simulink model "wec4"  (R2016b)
settings: Solver=ode4  StartTime=0  StopTime=1000  FixedStep=0.005  MaxStep=0.005  RelTol=1e-3  EnableMultiTasking=on
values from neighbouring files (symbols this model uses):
  arAdaptiveLawData = 1/2*zModelSimple.zModelPto.arFreq.*     zModelSimple.zModelPto.arMagnitude./     cos(zModelSimple.zModelPto.arPhase*pi/180+pi/2)    [IMPACT_Control.m]
  arAdaptiveLawDataX = 1/2*zModelSimpleX.zModelPto.arFreq.*         zModelSimpleX.zModelPto.arMagnitude./         cos(zModelSimpleX.zModelPto.arPhase*pi/180+pi/2)    [IMPACT_Control.m]
  arControllerRampGain = [0,0,1,1]    [IMPACT_Control.m]
  arControllerRampTime = [0 rStartRampTime rStartRampTime+rRampTimeLength 8000]    [IMPACT_Control.m]
  arEkfInitialisation = zeros(1,11)    [IMPACT_Control.m]
  arEkfInitialisationX = zeros(1,11)    [IMPACT_Control.m]
  arFrequency = zModelSimple.zModelPto.arFreq    [IMPACT_Control.m]
  arFrequencyRange = zModelSimple.zModelPto.arFreq    [IMPACT_Control.m]
  arFrequencyX = zModelSimpleX.zModelPto.arFreq    [IMPACT_Control.m]
  arImpedance = 1./zModelSimple.zModelPto.arMagnitude./zModelSimple.zModelPto.arFreq    [IMPACT_Control.m]
  arImpedanceX = 1./zModelSimpleX.zModelPto.arMagnitude./zModelSimpleX.zModelPto.arFreq    [IMPACT_Control.m]
  CentralPTOPreload = -1.6113e+07    (= -16113000)    [wecSimInputFile.m]
  F1 = [4.243 2.375 -12.243]    [wecSimInputFile.m]
  F2 = [4.243 -2.375 -12.243]    [wecSimInputFile.m]
  F3 = [-4.243 -2.375 -12.243]    [wecSimInputFile.m]
  F4 = [-4.243 2.375 -12.243]    [wecSimInputFile.m]
  FC = [0 0 -14]    [wecSimInputFile.m]
  iAdaptiveDamping = 0    [wec4IMPACT_Project.m]    (also in IMPACT_Control.m = handles.iAdaptiveDamping; wec1_IMPACT_Project.m; wec2_IMPACT_Project.m; wec3_IMPACT_Project.m)
  iControlType = 2    [wec4IMPACT_Project.m]    (also in IMPACT_Control.m = handles.iControlType; wec1_IMPACT_Project.m = 1; wec2_IMPACT_Project.m = 1; wec3_IMPACT_Project.m = 1)
  iPtoPositionConstraint = 1    [wec4IMPACT_Project.m]    (also in IMPACT_Control.m = handles.iPtoPositionConstraint; wec1_IMPACT_Project.m = 0; wec2_IMPACT_Project.m; wec3_IMPACT_Project.m)
  iSensorNoise = 0    [IMPACT_Control.m]
  m = m+1    (= 2)    [checkParamFile.m]
  PTOrotation = atan((T1(2)-F1(2))/(T1(1)-F1(1)))    [wecSimInputFile.m]
  rCogFloater = -8    [wec4_IMPACT_Model.m]    (also in paramInitial.m = get( handles.edit_rCogFloater, 'String' ); wec1_IMPACT_Model.m = -18; wec2_IMPACT_Model.m = -8.5; wec3_IMPACT_Model.m = -0.7)
  rCogSpar = -36.6    [wec4_IMPACT_Model.m]    (also in paramInitial.m = get( handles.edit_rCogSpar, 'String' ); wec3_IMPACT_Model.m = -21.3; wec3_IMPACT_Model2.m = -21.3)
  rDisplacementLimit = 10.000000    (= 10)    [wec4IMPACT_Project.m]    (also in IMPACT_Control.m = getValue(handles.edit_displacementLimit); wec1_IMPACT_Project.m; wec2_IMPACT_Project.m; wec3_IMPACT_Project.m = 3)
  rDisplacementLimitX = 10.000000    (= 10)    [wec4IMPACT_Project.m]    (also in IMPACT_Control.m = getValue(handles.edit_displacementLimitX); wec1_IMPACT_Project.m = 0; wec2_IMPACT_Project.m; wec3_IMPACT_Project.m = 0)
  rGainForAntiWIndUp = tfControllerDiscrete.rGain    [IMPACT_Control.m]
  rGainForAntiWIndUpX = tfControllerXDiscrete.rGain    [IMPACT_Control.m]
  rMaxForcePto = 300000000.000000    (= 300000000)    [wec4IMPACT_Project.m]    (also in IMPACT_Control.m = getValue(handles.edit_maxForcePto); wec1_IMPACT_Project.m = 1e+15; wec2_IMPACT_Project.m = 1e+15; wec3_IMPACT_Project.m = 1000000000)
  rMinForcePto = -300000000.000000    (= -300000000)    [wec4IMPACT_Project.m]    (also in IMPACT_Control.m = getValue(handles.edit_minForcePto); wec1_IMPACT_Project.m = -1e+15; wec2_IMPACT_Project.m = -1e+15; wec3_IMPACT_Project.m = -1000000000)
  rMooringX = 20000    [wec4_IMPACT_Model.m]    (also in paramInitial.m = get( handles.edit_rMooringX, 'String' ); wec3_IMPACT_Model.m = 10000; wec3_IMPACT_Model2.m = 10000)
  rMooringZ = 10000    [wec4_IMPACT_Model.m]    (also in paramInitial.m = get( handles.edit_rMooringZ, 'String' ); wec3_IMPACT_Model.m = 0; wec3_IMPACT_Model2.m = 0)
  rOutputSampleTime = 0.010000    (= 0.01)    [wec4IMPACT_Project.m]    (also in IMPACT_Control.m = getValue(handles.edit_outputSampleTime); wec1_IMPACT_Project.m; wec2_IMPACT_Project.m; wec3_IMPACT_Project.m)
  rPassiveDampingGain = -604830.000000    (= -604830)    [wec4IMPACT_Project.m]    (also in IMPACT_Control.m = getValue(handles.edit_gainPLD); wec1_IMPACT_Project.m = -214018.1537; wec2_IMPACT_Project.m = -1948070; wec3_IMPACT_Project.m = -519390)
  rPassiveDampingGainX = -278660.000000    (= -278660)    [wec4IMPACT_Project.m]    (also in IMPACT_Control.m = getValue(handles.edit_gainPLDX); wec1_IMPACT_Project.m = 0; wec2_IMPACT_Project.m = 0; wec3_IMPACT_Project.m = 0)
  rTetherPretension = 1.6113e+07    (= 16113000)    [wec4_IMPACT_Model.m]    (also in paramInitial.m = get( handles.edit_rTetherPretension, 'String' ); wec3_IMPACT_Model.m = 0; wec3_IMPACT_Model2.m = 0)
  rTetherSpring = 500000    [wec4_IMPACT_Model.m]    (also in paramInitial.m = get( handles.edit_rTetherSpring, 'String' ); wec3_IMPACT_Model.m = 0; wec3_IMPACT_Model2.m = 0)
  rUpperFrequencyLimit = EKFFloater.upperFreq    [IMPACT_Control.m]
  rXf = 4.243    [wec4AdditionalParams.m]
  rXs = 16.075    [wec4AdditionalParams.m]
  rYf = 2.375    [wec4AdditionalParams.m]
  rYs = 16.075    [wec4AdditionalParams.m]
  rZf = 4.243    [wec4AdditionalParams.m]
  rZs = 2.4350    (= 2.435)    [wec4AdditionalParams.m]
  rZTetherF = 6    [wec4AdditionalParams.m]
  rZTetherS = 2.4350    (= 2.435)    [wec4AdditionalParams.m]
  s = tf('s')    [wec4_IMPACT_Model.m]    (also in IMPACT_Control.m; wec1_IMPACT_Model.m; wec2_IMPACT_Model.m; wec3_IMPACT_Model.m)
  SidePTO1Preload = PreloadPTOCorner    (= 0)    [wecSimInputFile.m]
  SidePTO2Preload = PreloadPTOCorner    (= 0)    [wecSimInputFile.m]
  SidePTO3Preload = PreloadPTOCorner    (= 0)    [wecSimInputFile.m]
  SidePTO4Preload = PreloadPTOCorner    (= 0)    [wecSimInputFile.m]
  simu = simulationClass()    [wecSimInputFile.m]
  T1 = [16.075 16.075 -34.165]    [wecSimInputFile.m]
  T2 = [16.075 -16.075 -34.165]    [wecSimInputFile.m]
  T3 = [-16.075 -16.075 -34.165]    [wecSimInputFile.m]
  T4 = [-16.075 16.075 -34.165]    [wecSimInputFile.m]
  TC = [0 0 -34.165]    [wecSimInputFile.m]
  waves = waveClass('irregular')    [wecSimInputFile.m]
  Z = magPhaseToComplex(zModelTf)    [IMPACT_Control.m]
undefined symbols (not defined in the file or in its folder): arControllerDiscreteDen, arControllerDiscreteNum, arControllerDiscreteXDen, arControllerDiscreteXNum, arExcForceFloaterDen, arExcForceFloaterNum, arExcForceFloaterXDen, arExcForceFloaterXNum, arExcForceSparDen, arExcForceSparNum, arExcForceSparXDen, arExcForceSparXNum, arFexcFloaterDen, arFexcFloaterNum, arFexcFloaterXDen, arFexcFloaterXNum, arFexcSparDen, arFexcSparNum, arFexcSparXDen, arFexcSparXNum, Body, body, constraint, CTTime, deg, Elements, geometry, IRKB, kg, lenJ, mooring, N, pto, rAccelerationGainFloater, rAccelerationGainFloaterX, rAccelerationGainSpar, rAccelerationGainSparX, rad, rBuoyancyGainFloater, rBuoyancyGainFloaterX, rBuoyancyGainSpar, rBuoyancyGainSparX, rDampingGainFloater, rDampingGainFloaterX, rDampingGainSpar, rDampingGainSparX, Rigid, rMaxFocePto, wec4_float, wec4_reactor, WECSim_Lib, X, Y
libraries: nesl_utility x380, sm_lib x170, vrlib x91, simulink x12, WECSim_Lib x4
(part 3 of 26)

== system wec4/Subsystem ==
  Vel floater 6x1 : Inport
  Vel Spar 6x1 : Inport  Port=2
  Selector1 : Selector  InputPortWidth=6  IndexOptions=Index vector (dialog)  Indices=3  OutputSizes=1
  Selector18 : Selector  InputPortWidth=6  IndexOptions=Index vector (dialog)  Indices=1  OutputSizes=1
  Selector2 : Selector  InputPortWidth=6  IndexOptions=Index vector (dialog)  Indices=3  OutputSizes=1
  Selector3 : Selector  InputPortWidth=6  IndexOptions=Index vector (dialog)  Indices=1  OutputSizes=1
  Sum5 : Sum  Inputs=|+-
  Sum6 : Sum  Inputs=|+-
  "Rel. vel. X " : Outport
  Rel. vel. Z : Outport  Port=2
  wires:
  Selector1/1 -> Sum6/1
  Selector2/1 -> Sum6/2
  Vel floater 6x1/1 -> Selector1/1, Selector18/1
  Selector3/1 -> Sum5/2
  Vel Spar 6x1/1 -> Selector2/1, Selector3/1
  Selector18/1 -> Sum5/1
  Sum5/1 -> "Rel. vel. X "/1
  Sum6/1 -> Rel. vel. Z/1

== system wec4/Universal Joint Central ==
  Assignment : Assignment  DiagnosticForDimensions=Warning  IndexOptions=Index vector (dialog)  Indices=[4 5]  OutputSizes=1
  Assignment1 : Assignment  DiagnosticForDimensions=Warning  IndexOptions=Index vector (dialog)  Indices=[4 5]  OutputSizes=1
  Assignment2 : Assignment  DiagnosticForDimensions=Warning  IndexOptions=Index vector (dialog)  Indices=[4 5]  OutputSizes=1
  CONSTRAINT Universal Joint : sm_lib/Joints/Universal Joint  SenseConstraintForce=on  SenseConstraintForceX=off  SenseConstraintForceY=off  SenseConstraintForceZ=off  SenseConstraintTorque=on  SenseConstraintTorqueX=off  SenseConstraintTorqueY=off  SenseConstraintTorqueZ=off  SenseTotalForce=off  SenseTotalForceX=off  SenseTotalForceY=off  SenseTotalForceZ=off  SenseTotalTorque=off  SenseTotalTorqueX=off  SenseTotalTorqueY=off  SenseTotalTorqueZ=off  CompositeWrenchDir=BaseOnFollower  CompositeWrenchFrame=BaseFrame  RxEquilibriumPosition=0  RxEquilibriumPositionUnits=deg  RxSpringStiffness=0  RxSpringStiffnessUnits=N*m/deg  RxDampingCoefficient=0  RxDampingCoefficientUnits=N*m/(deg/s)  RxTorqueActuationMode=NoTorque  RxMotionActuationMode=ComputedMotion  RxSensePosition=on  RxSenseVelocity=on  RxSenseAcceleration=on  RxSenseTorqueForce=off  RxPositionTargetSpecify=off  RxPositionTargetPriority=High  RxPositionTargetValue=0  RxPositionTargetValueUnits=deg  RxVelocityTargetSpecify=off  RxVelocityTargetPriority=High  RxVelocityTargetValue=0  RxVelocityTargetValueUnits=deg/s  RyEquilibriumPosition=0  RyEquilibriumPositionUnits=deg  RySpringStiffness=0  RySpringStiffnessUnits=N*m/deg  RyDampingCoefficient=0  RyDampingCoefficientUnits=N*m/(deg/s)  RyTorqueActuationMode=NoTorque  RyMotionActuationMode=ComputedMotion  RySensePosition=on  RySenseVelocity=on  RySenseAcceleration=on  RySenseTorqueForce=off  RyPositionTargetSpecify=off  RyPositionTargetPriority=High  RyPositionTargetValue=0  RyPositionTargetValueUnits=deg  RyVelocityTargetSpecify=off  RyVelocityTargetPriority=High  RyVelocityTargetValue=0  RyVelocityTargetValueUnits=deg/s
  Constant : Constant  Value=[0 0 0 0 0 0]
  Constant1 : Constant  Value=[0 0 0 0 0 0]
  Constant2 : Constant  Value=[0 0 0 0 0 0]
  Mux{,2..4} (4 alike) : Mux  Inputs=2
  Mux1 : Mux
  PS-Simulink Converter{1..5,7,9,11} (8 alike) : nesl_utility/PS-Simulink Converter  PhysicalDomain=network_engine_domain  SubClassName=ps_output  LeftPortType=input  RightPortType=output  PseudoPeriodic=off  Frequencies=[]  Unit=1  AffineConversion=off
  Rigid Transform (Position) : sm_lib/Frames and Transforms/Rigid Transform  TranslationMethod=Cartesian  TranslationStandardOffset=0  TranslationLengthUnit=m  TranslationStandardAxis=+Z  TranslationCartesianOffset=constraint.initDisp.initLinDisp+constraint.loc  TranslationROffset=0  TranslationROffsetUnits=m  TranslationZOffset=0  TranslationZOffsetUnits=m  TranslationThetaOffset=0  TranslationThetaOffsetUnits=deg  RotationMethod=None  RotationAngleUnits=rad  RotationStandardAxis=+Y  RotationAngle=0  RotationArbitraryAxis=[0 1 0]  FollAlignAxisA=+X  BaseAlignAxisA=+Y  FollAlignAxisB=+Y  BaseAlignAxisB=+Z  RotationSequenceAxes=FollowerAxes  RotationSequence=XYX  RotationSequenceAngles=[0 0 0]  RotationSequenceAnglesUnits=deg  RotationMatrix=[1 0 0; 0 1 0; 0 0 1]
  Rigid Transform (Position)1 : sm_lib/Frames and Transforms/Rigid Transform  TranslationMethod=Cartesian  TranslationStandardOffset=0  TranslationLengthUnit=m  TranslationStandardAxis=+Z  TranslationCartesianOffset=constraint.initDisp.initLinDisp+constraint.loc  TranslationROffset=0  TranslationROffsetUnits=m  TranslationZOffset=0  TranslationZOffsetUnits=m  TranslationThetaOffset=0  TranslationThetaOffsetUnits=deg  RotationMethod=None  RotationAngleUnits=rad  RotationStandardAxis=+Y  RotationAngle=0  RotationArbitraryAxis=[0 1 0]  FollAlignAxisA=+X  BaseAlignAxisA=+Y  FollAlignAxisB=+Y  BaseAlignAxisB=+Z  RotationSequenceAxes=FollowerAxes  RotationSequence=XYX  RotationSequenceAngles=[0 0 0]  RotationSequenceAnglesUnits=deg  RotationMatrix=[1 0 0; 0 1 0; 0 0 1]
  Rigid Transform (Orientation) : sm_lib/Frames and Transforms/Rigid Transform  TranslationMethod=None  TranslationStandardOffset=0  TranslationLengthUnit=m  TranslationStandardAxis=+Z  TranslationCartesianOffset=constraint.loc  TranslationROffset=0  TranslationROffsetUnits=m  TranslationZOffset=0  TranslationZOffsetUnits=m  TranslationThetaOffset=0  TranslationThetaOffsetUnits=deg  RotationMethod=RotationMatrix  RotationAngleUnits=rad  RotationStandardAxis=+Y  RotationAngle=0  RotationArbitraryAxis=[0 1 0]  FollAlignAxisA=+X  BaseAlignAxisA=+Y  FollAlignAxisB=+Y  BaseAlignAxisB=+Z  RotationSequenceAxes=FollowerAxes  RotationSequence=XYX  RotationSequenceAngles=[0 0 0]  RotationSequenceAnglesUnits=deg  RotationMatrix=constraint.orientation.rotationMatrix
  Rigid Transform (Orientation)1 : sm_lib/Frames and Transforms/Rigid Transform  TranslationMethod=None  TranslationStandardOffset=0  TranslationLengthUnit=m  TranslationStandardAxis=+Z  TranslationCartesianOffset=constraint.loc  TranslationROffset=0  TranslationROffsetUnits=m  TranslationZOffset=0  TranslationZOffsetUnits=m  TranslationThetaOffset=0  TranslationThetaOffsetUnits=deg  RotationMethod=RotationMatrix  RotationAngleUnits=rad  RotationStandardAxis=+Y  RotationAngle=0  RotationArbitraryAxis=[0 1 0]  FollAlignAxisA=+X  BaseAlignAxisA=+Y  FollAlignAxisB=+Y  BaseAlignAxisB=+Z  RotationSequenceAxes=FollowerAxes  RotationSequence=XYX  RotationSequenceAngles=[0 0 0]  RotationSequenceAnglesUnits=deg  RotationMatrix=constraint.orientation.rotationMatrix
  output : ToWorkspace  VariableName=constraint2_out  SaveFormat=Structure With Time  SampleTime=-1
  F : PMIOPort  Port=1  Side=Right
  B : PMIOPort  Port=2  Side=Left
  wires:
  PS-Simulink Converter4/1 -> Mux/2
  PS-Simulink Converter3/1 -> Mux/1
  Mux3/1 -> Assignment1/2
  Mux4/1 -> Assignment/2
  Constant/1 -> Assignment/1
  Constant1/1 -> Assignment1/1
  Constant2/1 -> Assignment2/1
  Assignment2/1 -> Mux1/3  "acceleration"
  Assignment1/1 -> Mux1/2  "velocity"
  Assignment/1 -> Mux1/1  "position"
  Mux/1 -> Mux1/4  "Constraint Forces"
  Mux1/1 -> output/1
  PS-Simulink Converter5/1 -> Mux2/2
  Mux2/1 -> Assignment2/2
  PS-Simulink Converter2/1 -> Mux3/2
  PS-Simulink Converter9/1 -> Mux3/1
  PS-Simulink Converter11/1 -> Mux4/2
  PS-Simulink Converter1/1 -> Mux4/1
  PS-Simulink Converter7/1 -> Mux2/1
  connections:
  Rigid Transform (Position)1/LConn1 -- F/RConn1
  Rigid Transform (Position)1/RConn1 -- Rigid Transform (Orientation)1/LConn1
  Rigid Transform (Orientation)/RConn1 -- CONSTRAINT Universal Joint/LConn1
  Rigid Transform (Position)/RConn1 -- Rigid Transform (Orientation)/LConn1
  Rigid Transform (Position)/LConn1 -- B/RConn1
  CONSTRAINT Universal Joint/RConn8 -- PS-Simulink Converter3/LConn1
  PS-Simulink Converter4/LConn1 -- CONSTRAINT Universal Joint/RConn9
  PS-Simulink Converter1/LConn1 -- CONSTRAINT Universal Joint/RConn2
  PS-Simulink Converter11/LConn1 -- CONSTRAINT Universal Joint/RConn5
  PS-Simulink Converter9/LConn1 -- CONSTRAINT Universal Joint/RConn3
  PS-Simulink Converter7/LConn1 -- CONSTRAINT Universal Joint/RConn4
  PS-Simulink Converter2/LConn1 -- CONSTRAINT Universal Joint/RConn6
  PS-Simulink Converter5/LConn1 -- CONSTRAINT Universal Joint/RConn7
  CONSTRAINT Universal Joint/RConn1 -- Rigid Transform (Orientation)1/RConn1

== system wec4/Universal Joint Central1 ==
  Assignment : Assignment  DiagnosticForDimensions=Warning  IndexOptions=Index vector (dialog)  Indices=[4 5]  OutputSizes=1
  Assignment1 : Assignment  DiagnosticForDimensions=Warning  IndexOptions=Index vector (dialog)  Indices=[4 5]  OutputSizes=1
  Assignment2 : Assignment  DiagnosticForDimensions=Warning  IndexOptions=Index vector (dialog)  Indices=[4 5]  OutputSizes=1
  CONSTRAINT Universal Joint : sm_lib/Joints/Universal Joint  SenseConstraintForce=on  SenseConstraintForceX=off  SenseConstraintForceY=off  SenseConstraintForceZ=off  SenseConstraintTorque=on  SenseConstraintTorqueX=off  SenseConstraintTorqueY=off  SenseConstraintTorqueZ=off  SenseTotalForce=off  SenseTotalForceX=off  SenseTotalForceY=off  SenseTotalForceZ=off  SenseTotalTorque=off  SenseTotalTorqueX=off  SenseTotalTorqueY=off  SenseTotalTorqueZ=off  CompositeWrenchDir=BaseOnFollower  CompositeWrenchFrame=BaseFrame  RxEquilibriumPosition=0  RxEquilibriumPositionUnits=deg  RxSpringStiffness=0  RxSpringStiffnessUnits=N*m/deg  RxDampingCoefficient=0  RxDampingCoefficientUnits=N*m/(deg/s)  RxTorqueActuationMode=NoTorque  RxMotionActuationMode=ComputedMotion  RxSensePosition=on  RxSenseVelocity=on  RxSenseAcceleration=on  RxSenseTorqueForce=off  RxPositionTargetSpecify=off  RxPositionTargetPriority=High  RxPositionTargetValue=0  RxPositionTargetValueUnits=deg  RxVelocityTargetSpecify=off  RxVelocityTargetPriority=High  RxVelocityTargetValue=0  RxVelocityTargetValueUnits=deg/s  RyEquilibriumPosition=0  RyEquilibriumPositionUnits=deg  RySpringStiffness=0  RySpringStiffnessUnits=N*m/deg  RyDampingCoefficient=0  RyDampingCoefficientUnits=N*m/(deg/s)  RyTorqueActuationMode=NoTorque  RyMotionActuationMode=ComputedMotion  RySensePosition=on  RySenseVelocity=on  RySenseAcceleration=on  RySenseTorqueForce=off  RyPositionTargetSpecify=off  RyPositionTargetPriority=High  RyPositionTargetValue=0  RyPositionTargetValueUnits=deg  RyVelocityTargetSpecify=off  RyVelocityTargetPriority=High  RyVelocityTargetValue=0  RyVelocityTargetValueUnits=deg/s
  Constant : Constant  Value=[0 0 0 0 0 0]
  Constant1 : Constant  Value=[0 0 0 0 0 0]
  Constant2 : Constant  Value=[0 0 0 0 0 0]
  Mux{,2..4} (4 alike) : Mux  Inputs=2
  Mux1 : Mux
  PS-Simulink Converter{1..5,7,9,11} (8 alike) : nesl_utility/PS-Simulink Converter  PhysicalDomain=network_engine_domain  SubClassName=ps_output  LeftPortType=input  RightPortType=output  PseudoPeriodic=off  Frequencies=[]  Unit=1  AffineConversion=off
  Rigid Transform (Position) : sm_lib/Frames and Transforms/Rigid Transform  TranslationMethod=Cartesian  TranslationStandardOffset=0  TranslationLengthUnit=m  TranslationStandardAxis=+Z  TranslationCartesianOffset=constraint.initDisp.initLinDisp+constraint.loc  TranslationROffset=0  TranslationROffsetUnits=m  TranslationZOffset=0  TranslationZOffsetUnits=m  TranslationThetaOffset=0  TranslationThetaOffsetUnits=deg  RotationMethod=None  RotationAngleUnits=rad  RotationStandardAxis=+Y  RotationAngle=0  RotationArbitraryAxis=[0 1 0]  FollAlignAxisA=+X  BaseAlignAxisA=+Y  FollAlignAxisB=+Y  BaseAlignAxisB=+Z  RotationSequenceAxes=FollowerAxes  RotationSequence=XYX  RotationSequenceAngles=[0 0 0]  RotationSequenceAnglesUnits=deg  RotationMatrix=[1 0 0; 0 1 0; 0 0 1]
  Rigid Transform (Position)1 : sm_lib/Frames and Transforms/Rigid Transform  TranslationMethod=Cartesian  TranslationStandardOffset=0  TranslationLengthUnit=m  TranslationStandardAxis=+Z  TranslationCartesianOffset=constraint.initDisp.initLinDisp+constraint.loc  TranslationROffset=0  TranslationROffsetUnits=m  TranslationZOffset=0  TranslationZOffsetUnits=m  TranslationThetaOffset=0  TranslationThetaOffsetUnits=deg  RotationMethod=None  RotationAngleUnits=rad  RotationStandardAxis=+Y  RotationAngle=0  RotationArbitraryAxis=[0 1 0]  FollAlignAxisA=+X  BaseAlignAxisA=+Y  FollAlignAxisB=+Y  BaseAlignAxisB=+Z  RotationSequenceAxes=FollowerAxes  RotationSequence=XYX  RotationSequenceAngles=[0 0 0]  RotationSequenceAnglesUnits=deg  RotationMatrix=[1 0 0; 0 1 0; 0 0 1]
  Rigid Transform (Orientation) : sm_lib/Frames and Transforms/Rigid Transform  TranslationMethod=None  TranslationStandardOffset=0  TranslationLengthUnit=m  TranslationStandardAxis=+Z  TranslationCartesianOffset=constraint.loc  TranslationROffset=0  TranslationROffsetUnits=m  TranslationZOffset=0  TranslationZOffsetUnits=m  TranslationThetaOffset=0  TranslationThetaOffsetUnits=deg  RotationMethod=RotationMatrix  RotationAngleUnits=rad  RotationStandardAxis=+Y  RotationAngle=0  RotationArbitraryAxis=[0 1 0]  FollAlignAxisA=+X  BaseAlignAxisA=+Y  FollAlignAxisB=+Y  BaseAlignAxisB=+Z  RotationSequenceAxes=FollowerAxes  RotationSequence=XYX  RotationSequenceAngles=[0 0 0]  RotationSequenceAnglesUnits=deg  RotationMatrix=constraint.orientation.rotationMatrix
  Rigid Transform (Orientation)1 : sm_lib/Frames and Transforms/Rigid Transform  TranslationMethod=None  TranslationStandardOffset=0  TranslationLengthUnit=m  TranslationStandardAxis=+Z  TranslationCartesianOffset=constraint.loc  TranslationROffset=0  TranslationROffsetUnits=m  TranslationZOffset=0  TranslationZOffsetUnits=m  TranslationThetaOffset=0  TranslationThetaOffsetUnits=deg  RotationMethod=RotationMatrix  RotationAngleUnits=rad  RotationStandardAxis=+Y  RotationAngle=0  RotationArbitraryAxis=[0 1 0]  FollAlignAxisA=+X  BaseAlignAxisA=+Y  FollAlignAxisB=+Y  BaseAlignAxisB=+Z  RotationSequenceAxes=FollowerAxes  RotationSequence=XYX  RotationSequenceAngles=[0 0 0]  RotationSequenceAnglesUnits=deg  RotationMatrix=constraint.orientation.rotationMatrix
  output : ToWorkspace  VariableName=constraint3_out  SaveFormat=Structure With Time  SampleTime=-1
  F : PMIOPort  Port=1  Side=Right
  B : PMIOPort  Port=2  Side=Left
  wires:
  PS-Simulink Converter4/1 -> Mux/2
  PS-Simulink Converter3/1 -> Mux/1
  Mux3/1 -> Assignment1/2
  Mux4/1 -> Assignment/2
  Constant/1 -> Assignment/1
  Constant1/1 -> Assignment1/1
  Constant2/1 -> Assignment2/1
  Assignment2/1 -> Mux1/3  "acceleration"
  Assignment1/1 -> Mux1/2  "velocity"
  Assignment/1 -> Mux1/1  "position"
  Mux/1 -> Mux1/4  "Constraint Forces"
  Mux1/1 -> output/1
  PS-Simulink Converter5/1 -> Mux2/2
  Mux2/1 -> Assignment2/2
  PS-Simulink Converter2/1 -> Mux3/2
  PS-Simulink Converter9/1 -> Mux3/1
  PS-Simulink Converter11/1 -> Mux4/2
  PS-Simulink Converter1/1 -> Mux4/1
  PS-Simulink Converter7/1 -> Mux2/1
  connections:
  Rigid Transform (Position)1/LConn1 -- F/RConn1
  Rigid Transform (Position)1/RConn1 -- Rigid Transform (Orientation)1/LConn1
  Rigid Transform (Orientation)/RConn1 -- CONSTRAINT Universal Joint/LConn1
  Rigid Transform (Position)/RConn1 -- Rigid Transform (Orientation)/LConn1
  Rigid Transform (Position)/LConn1 -- B/RConn1
  CONSTRAINT Universal Joint/RConn8 -- PS-Simulink Converter3/LConn1
  PS-Simulink Converter4/LConn1 -- CONSTRAINT Universal Joint/RConn9
  PS-Simulink Converter1/LConn1 -- CONSTRAINT Universal Joint/RConn2
  PS-Simulink Converter11/LConn1 -- CONSTRAINT Universal Joint/RConn5
  PS-Simulink Converter9/LConn1 -- CONSTRAINT Universal Joint/RConn3
  PS-Simulink Converter7/LConn1 -- CONSTRAINT Universal Joint/RConn4
  PS-Simulink Converter2/LConn1 -- CONSTRAINT Universal Joint/RConn6
  PS-Simulink Converter5/LConn1 -- CONSTRAINT Universal Joint/RConn7
  CONSTRAINT Universal Joint/RConn1 -- Rigid Transform (Orientation)1/RConn1

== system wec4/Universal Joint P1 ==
  Assignment : Assignment  DiagnosticForDimensions=Warning  IndexOptions=Index vector (dialog)  Indices=[4 5]  OutputSizes=1
  Assignment1 : Assignment  DiagnosticForDimensions=Warning  IndexOptions=Index vector (dialog)  Indices=[4 5]  OutputSizes=1
  Assignment2 : Assignment  DiagnosticForDimensions=Warning  IndexOptions=Index vector (dialog)  Indices=[4 5]  OutputSizes=1
  CONSTRAINT Universal Joint : sm_lib/Joints/Universal Joint  SenseConstraintForce=on  SenseConstraintForceX=off  SenseConstraintForceY=off  SenseConstraintForceZ=off  SenseConstraintTorque=on  SenseConstraintTorqueX=off  SenseConstraintTorqueY=off  SenseConstraintTorqueZ=off  SenseTotalForce=off  SenseTotalForceX=off  SenseTotalForceY=off  SenseTotalForceZ=off  SenseTotalTorque=off  SenseTotalTorqueX=off  SenseTotalTorqueY=off  SenseTotalTorqueZ=off  CompositeWrenchDir=BaseOnFollower  CompositeWrenchFrame=BaseFrame  RxEquilibriumPosition=0  RxEquilibriumPositionUnits=deg  RxSpringStiffness=0  RxSpringStiffnessUnits=N*m/deg  RxDampingCoefficient=0  RxDampingCoefficientUnits=N*m/(deg/s)  RxTorqueActuationMode=NoTorque  RxMotionActuationMode=ComputedMotion  RxSensePosition=on  RxSenseVelocity=on  RxSenseAcceleration=on  RxSenseTorqueForce=off  RxPositionTargetSpecify=off  RxPositionTargetPriority=High  RxPositionTargetValue=0  RxPositionTargetValueUnits=deg  RxVelocityTargetSpecify=off  RxVelocityTargetPriority=High  RxVelocityTargetValue=0  RxVelocityTargetValueUnits=deg/s  RyEquilibriumPosition=0  RyEquilibriumPositionUnits=deg  RySpringStiffness=0  RySpringStiffnessUnits=N*m/deg  RyDampingCoefficient=0  RyDampingCoefficientUnits=N*m/(deg/s)  RyTorqueActuationMode=NoTorque  RyMotionActuationMode=ComputedMotion  RySensePosition=on  RySenseVelocity=on  RySenseAcceleration=on  RySenseTorqueForce=off  RyPositionTargetSpecify=off  RyPositionTargetPriority=High  RyPositionTargetValue=0  RyPositionTargetValueUnits=deg  RyVelocityTargetSpecify=off  RyVelocityTargetPriority=High  RyVelocityTargetValue=0  RyVelocityTargetValueUnits=deg/s
  Constant : Constant  Value=[0 0 0 0 0 0]
  Constant1 : Constant  Value=[0 0 0 0 0 0]
  Constant2 : Constant  Value=[0 0 0 0 0 0]
  Mux{,2..4} (4 alike) : Mux  Inputs=2
  Mux1 : Mux
  PS-Simulink Converter{1..5,7,9,11} (8 alike) : nesl_utility/PS-Simulink Converter  PhysicalDomain=network_engine_domain  SubClassName=ps_output  LeftPortType=input  RightPortType=output  PseudoPeriodic=off  Frequencies=[]  Unit=1  AffineConversion=off
  Rigid Transform (Position) : sm_lib/Frames and Transforms/Rigid Transform  TranslationMethod=Cartesian  TranslationStandardOffset=0  TranslationLengthUnit=m  TranslationStandardAxis=+Z  TranslationCartesianOffset=constraint.initDisp.initLinDisp+constraint.loc  TranslationROffset=0  TranslationROffsetUnits=m  TranslationZOffset=0  TranslationZOffsetUnits=m  TranslationThetaOffset=0  TranslationThetaOffsetUnits=deg  RotationMethod=None  RotationAngleUnits=rad  RotationStandardAxis=+Y  RotationAngle=0  RotationArbitraryAxis=[0 1 0]  FollAlignAxisA=+X  BaseAlignAxisA=+Y  FollAlignAxisB=+Y  BaseAlignAxisB=+Z  RotationSequenceAxes=FollowerAxes  RotationSequence=XYX  RotationSequenceAngles=[0 0 0]  RotationSequenceAnglesUnits=deg  RotationMatrix=[1 0 0; 0 1 0; 0 0 1]
  Rigid Transform (Position)1 : sm_lib/Frames and Transforms/Rigid Transform  TranslationMethod=Cartesian  TranslationStandardOffset=0  TranslationLengthUnit=m  TranslationStandardAxis=+Z  TranslationCartesianOffset=constraint.initDisp.initLinDisp+constraint.loc  TranslationROffset=0  TranslationROffsetUnits=m  TranslationZOffset=0  TranslationZOffsetUnits=m  TranslationThetaOffset=0  TranslationThetaOffsetUnits=deg  RotationMethod=None  RotationAngleUnits=rad  RotationStandardAxis=+Y  RotationAngle=0  RotationArbitraryAxis=[0 1 0]  FollAlignAxisA=+X  BaseAlignAxisA=+Y  FollAlignAxisB=+Y  BaseAlignAxisB=+Z  RotationSequenceAxes=FollowerAxes  RotationSequence=XYX  RotationSequenceAngles=[0 0 0]  RotationSequenceAnglesUnits=deg  RotationMatrix=[1 0 0; 0 1 0; 0 0 1]
  Rigid Transform (Orientation) : sm_lib/Frames and Transforms/Rigid Transform  TranslationMethod=None  TranslationStandardOffset=0  TranslationLengthUnit=m  TranslationStandardAxis=+Z  TranslationCartesianOffset=constraint.loc  TranslationROffset=0  TranslationROffsetUnits=m  TranslationZOffset=0  TranslationZOffsetUnits=m  TranslationThetaOffset=0  TranslationThetaOffsetUnits=deg  RotationMethod=RotationMatrix  RotationAngleUnits=rad  RotationStandardAxis=+Y  RotationAngle=0  RotationArbitraryAxis=[0 1 0]  FollAlignAxisA=+X  BaseAlignAxisA=+Y  FollAlignAxisB=+Y  BaseAlignAxisB=+Z  RotationSequenceAxes=FollowerAxes  RotationSequence=XYX  RotationSequenceAngles=[0 0 0]  RotationSequenceAnglesUnits=deg  RotationMatrix=constraint.orientation.rotationMatrix
  Rigid Transform (Orientation)1 : sm_lib/Frames and Transforms/Rigid Transform  TranslationMethod=None  TranslationStandardOffset=0  TranslationLengthUnit=m  TranslationStandardAxis=+Z  TranslationCartesianOffset=constraint.loc  TranslationROffset=0  TranslationROffsetUnits=m  TranslationZOffset=0  TranslationZOffsetUnits=m  TranslationThetaOffset=0  TranslationThetaOffsetUnits=deg  RotationMethod=RotationMatrix  RotationAngleUnits=rad  RotationStandardAxis=+Y  RotationAngle=0  RotationArbitraryAxis=[0 1 0]  FollAlignAxisA=+X  BaseAlignAxisA=+Y  FollAlignAxisB=+Y  BaseAlignAxisB=+Z  RotationSequenceAxes=FollowerAxes  RotationSequence=XYX  RotationSequenceAngles=[0 0 0]  RotationSequenceAnglesUnits=deg  RotationMatrix=constraint.orientation.rotationMatrix
  output : ToWorkspace  VariableName=constraint4_out  SaveFormat=Structure With Time  SampleTime=-1
  F : PMIOPort  Port=1  Side=Right
  B : PMIOPort  Port=2  Side=Left
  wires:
  PS-Simulink Converter4/1 -> Mux/2
  PS-Simulink Converter3/1 -> Mux/1
  Mux3/1 -> Assignment1/2
  Mux4/1 -> Assignment/2
  Constant/1 -> Assignment/1
  Constant1/1 -> Assignment1/1
  Constant2/1 -> Assignment2/1
  Assignment2/1 -> Mux1/3  "acceleration"
  Assignment1/1 -> Mux1/2  "velocity"
  Assignment/1 -> Mux1/1  "position"
  Mux/1 -> Mux1/4  "Constraint Forces"
  Mux1/1 -> output/1
  PS-Simulink Converter5/1 -> Mux2/2
  Mux2/1 -> Assignment2/2
  PS-Simulink Converter2/1 -> Mux3/2
  PS-Simulink Converter9/1 -> Mux3/1
  PS-Simulink Converter11/1 -> Mux4/2
  PS-Simulink Converter1/1 -> Mux4/1
  PS-Simulink Converter7/1 -> Mux2/1
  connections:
  Rigid Transform (Position)1/LConn1 -- F/RConn1
  Rigid Transform (Position)1/RConn1 -- Rigid Transform (Orientation)1/LConn1
  Rigid Transform (Orientation)/RConn1 -- CONSTRAINT Universal Joint/LConn1
  Rigid Transform (Position)/RConn1 -- Rigid Transform (Orientation)/LConn1
  Rigid Transform (Position)/LConn1 -- B/RConn1
  CONSTRAINT Universal Joint/RConn8 -- PS-Simulink Converter3/LConn1
  PS-Simulink Converter4/LConn1 -- CONSTRAINT Universal Joint/RConn9
  PS-Simulink Converter1/LConn1 -- CONSTRAINT Universal Joint/RConn2
  PS-Simulink Converter11/LConn1 -- CONSTRAINT Universal Joint/RConn5
  PS-Simulink Converter9/LConn1 -- CONSTRAINT Universal Joint/RConn3
  PS-Simulink Converter7/LConn1 -- CONSTRAINT Universal Joint/RConn4
  PS-Simulink Converter2/LConn1 -- CONSTRAINT Universal Joint/RConn6
  PS-Simulink Converter5/LConn1 -- CONSTRAINT Universal Joint/RConn7
  CONSTRAINT Universal Joint/RConn1 -- Rigid Transform (Orientation)1/RConn1

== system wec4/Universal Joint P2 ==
  Assignment : Assignment  DiagnosticForDimensions=Warning  IndexOptions=Index vector (dialog)  Indices=[4 5]  OutputSizes=1
  Assignment1 : Assignment  DiagnosticForDimensions=Warning  IndexOptions=Index vector (dialog)  Indices=[4 5]  OutputSizes=1
  Assignment2 : Assignment  DiagnosticForDimensions=Warning  IndexOptions=Index vector (dialog)  Indices=[4 5]  OutputSizes=1
  CONSTRAINT Universal Joint : sm_lib/Joints/Universal Joint  SenseConstraintForce=on  SenseConstraintForceX=off  SenseConstraintForceY=off  SenseConstraintForceZ=off  SenseConstraintTorque=on  SenseConstraintTorqueX=off  SenseConstraintTorqueY=off  SenseConstraintTorqueZ=off  SenseTotalForce=off  SenseTotalForceX=off  SenseTotalForceY=off  SenseTotalForceZ=off  SenseTotalTorque=off  SenseTotalTorqueX=off  SenseTotalTorqueY=off  SenseTotalTorqueZ=off  CompositeWrenchDir=BaseOnFollower  CompositeWrenchFrame=BaseFrame  RxEquilibriumPosition=0  RxEquilibriumPositionUnits=deg  RxSpringStiffness=0  RxSpringStiffnessUnits=N*m/deg  RxDampingCoefficient=0  RxDampingCoefficientUnits=N*m/(deg/s)  RxTorqueActuationMode=NoTorque  RxMotionActuationMode=ComputedMotion  RxSensePosition=on  RxSenseVelocity=on  RxSenseAcceleration=on  RxSenseTorqueForce=off  RxPositionTargetSpecify=off  RxPositionTargetPriority=High  RxPositionTargetValue=0  RxPositionTargetValueUnits=deg  RxVelocityTargetSpecify=off  RxVelocityTargetPriority=High  RxVelocityTargetValue=0  RxVelocityTargetValueUnits=deg/s  RyEquilibriumPosition=0  RyEquilibriumPositionUnits=deg  RySpringStiffness=0  RySpringStiffnessUnits=N*m/deg  RyDampingCoefficient=0  RyDampingCoefficientUnits=N*m/(deg/s)  RyTorqueActuationMode=NoTorque  RyMotionActuationMode=ComputedMotion  RySensePosition=on  RySenseVelocity=on  RySenseAcceleration=on  RySenseTorqueForce=off  RyPositionTargetSpecify=off  RyPositionTargetPriority=High  RyPositionTargetValue=0  RyPositionTargetValueUnits=deg  RyVelocityTargetSpecify=off  RyVelocityTargetPriority=High  RyVelocityTargetValue=0  RyVelocityTargetValueUnits=deg/s
  Constant : Constant  Value=[0 0 0 0 0 0]
  Constant1 : Constant  Value=[0 0 0 0 0 0]
  Constant2 : Constant  Value=[0 0 0 0 0 0]
  Mux{,2..4} (4 alike) : Mux  Inputs=2
  Mux1 : Mux
  PS-Simulink Converter{1..5,7,9,11} (8 alike) : nesl_utility/PS-Simulink Converter  PhysicalDomain=network_engine_domain  SubClassName=ps_output  LeftPortType=input  RightPortType=output  PseudoPeriodic=off  Frequencies=[]  Unit=1  AffineConversion=off
  Rigid Transform (Position) : sm_lib/Frames and Transforms/Rigid Transform  TranslationMethod=Cartesian  TranslationStandardOffset=0  TranslationLengthUnit=m  TranslationStandardAxis=+Z  TranslationCartesianOffset=constraint.initDisp.initLinDisp+constraint.loc  TranslationROffset=0  TranslationROffsetUnits=m  TranslationZOffset=0  TranslationZOffsetUnits=m  TranslationThetaOffset=0  TranslationThetaOffsetUnits=deg  RotationMethod=None  RotationAngleUnits=rad  RotationStandardAxis=+Y  RotationAngle=0  RotationArbitraryAxis=[0 1 0]  FollAlignAxisA=+X  BaseAlignAxisA=+Y  FollAlignAxisB=+Y  BaseAlignAxisB=+Z  RotationSequenceAxes=FollowerAxes  RotationSequence=XYX  RotationSequenceAngles=[0 0 0]  RotationSequenceAnglesUnits=deg  RotationMatrix=[1 0 0; 0 1 0; 0 0 1]
  Rigid Transform (Position)1 : sm_lib/Frames and Transforms/Rigid Transform  TranslationMethod=Cartesian  TranslationStandardOffset=0  TranslationLengthUnit=m  TranslationStandardAxis=+Z  TranslationCartesianOffset=constraint.initDisp.initLinDisp+constraint.loc  TranslationROffset=0  TranslationROffsetUnits=m  TranslationZOffset=0  TranslationZOffsetUnits=m  TranslationThetaOffset=0  TranslationThetaOffsetUnits=deg  RotationMethod=None  RotationAngleUnits=rad  RotationStandardAxis=+Y  RotationAngle=0  RotationArbitraryAxis=[0 1 0]  FollAlignAxisA=+X  BaseAlignAxisA=+Y  FollAlignAxisB=+Y  BaseAlignAxisB=+Z  RotationSequenceAxes=FollowerAxes  RotationSequence=XYX  RotationSequenceAngles=[0 0 0]  RotationSequenceAnglesUnits=deg  RotationMatrix=[1 0 0; 0 1 0; 0 0 1]
  Rigid Transform (Orientation) : sm_lib/Frames and Transforms/Rigid Transform  TranslationMethod=None  TranslationStandardOffset=0  TranslationLengthUnit=m  TranslationStandardAxis=+Z  TranslationCartesianOffset=constraint.loc  TranslationROffset=0  TranslationROffsetUnits=m  TranslationZOffset=0  TranslationZOffsetUnits=m  TranslationThetaOffset=0  TranslationThetaOffsetUnits=deg  RotationMethod=RotationMatrix  RotationAngleUnits=rad  RotationStandardAxis=+Y  RotationAngle=0  RotationArbitraryAxis=[0 1 0]  FollAlignAxisA=+X  BaseAlignAxisA=+Y  FollAlignAxisB=+Y  BaseAlignAxisB=+Z  RotationSequenceAxes=FollowerAxes  RotationSequence=XYX  RotationSequenceAngles=[0 0 0]  RotationSequenceAnglesUnits=deg  RotationMatrix=constraint.orientation.rotationMatrix
  Rigid Transform (Orientation)1 : sm_lib/Frames and Transforms/Rigid Transform  TranslationMethod=None  TranslationStandardOffset=0  TranslationLengthUnit=m  TranslationStandardAxis=+Z  TranslationCartesianOffset=constraint.loc  TranslationROffset=0  TranslationROffsetUnits=m  TranslationZOffset=0  TranslationZOffsetUnits=m  TranslationThetaOffset=0  TranslationThetaOffsetUnits=deg  RotationMethod=RotationMatrix  RotationAngleUnits=rad  RotationStandardAxis=+Y  RotationAngle=0  RotationArbitraryAxis=[0 1 0]  FollAlignAxisA=+X  BaseAlignAxisA=+Y  FollAlignAxisB=+Y  BaseAlignAxisB=+Z  RotationSequenceAxes=FollowerAxes  RotationSequence=XYX  RotationSequenceAngles=[0 0 0]  RotationSequenceAnglesUnits=deg  RotationMatrix=constraint.orientation.rotationMatrix
  output : ToWorkspace  VariableName=constraint6_out  SaveFormat=Structure With Time  SampleTime=-1
  F : PMIOPort  Port=1  Side=Right
  B : PMIOPort  Port=2  Side=Left
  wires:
  PS-Simulink Converter4/1 -> Mux/2
  PS-Simulink Converter3/1 -> Mux/1
  Mux3/1 -> Assignment1/2
  Mux4/1 -> Assignment/2
  Constant/1 -> Assignment/1
  Constant1/1 -> Assignment1/1
  Constant2/1 -> Assignment2/1
  Assignment2/1 -> Mux1/3  "acceleration"
  Assignment1/1 -> Mux1/2  "velocity"
  Assignment/1 -> Mux1/1  "position"
  Mux/1 -> Mux1/4  "Constraint Forces"
  Mux1/1 -> output/1
  PS-Simulink Converter5/1 -> Mux2/2
  Mux2/1 -> Assignment2/2
  PS-Simulink Converter2/1 -> Mux3/2
  PS-Simulink Converter9/1 -> Mux3/1
  PS-Simulink Converter11/1 -> Mux4/2
  PS-Simulink Converter1/1 -> Mux4/1
  PS-Simulink Converter7/1 -> Mux2/1
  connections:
  Rigid Transform (Position)1/LConn1 -- F/RConn1
  Rigid Transform (Position)1/RConn1 -- Rigid Transform (Orientation)1/LConn1
  Rigid Transform (Orientation)/RConn1 -- CONSTRAINT Universal Joint/LConn1
  Rigid Transform (Position)/RConn1 -- Rigid Transform (Orientation)/LConn1
  Rigid Transform (Position)/LConn1 -- B/RConn1
  CONSTRAINT Universal Joint/RConn8 -- PS-Simulink Converter3/LConn1
  PS-Simulink Converter4/LConn1 -- CONSTRAINT Universal Joint/RConn9
  PS-Simulink Converter1/LConn1 -- CONSTRAINT Universal Joint/RConn2
  PS-Simulink Converter11/LConn1 -- CONSTRAINT Universal Joint/RConn5
  PS-Simulink Converter9/LConn1 -- CONSTRAINT Universal Joint/RConn3
  PS-Simulink Converter7/LConn1 -- CONSTRAINT Universal Joint/RConn4
  PS-Simulink Converter2/LConn1 -- CONSTRAINT Universal Joint/RConn6
  PS-Simulink Converter5/LConn1 -- CONSTRAINT Universal Joint/RConn7
  CONSTRAINT Universal Joint/RConn1 -- Rigid Transform (Orientation)1/RConn1

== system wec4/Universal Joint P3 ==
  Assignment : Assignment  DiagnosticForDimensions=Warning  IndexOptions=Index vector (dialog)  Indices=[4 5]  OutputSizes=1
  Assignment1 : Assignment  DiagnosticForDimensions=Warning  IndexOptions=Index vector (dialog)  Indices=[4 5]  OutputSizes=1
  Assignment2 : Assignment  DiagnosticForDimensions=Warning  IndexOptions=Index vector (dialog)  Indices=[4 5]  OutputSizes=1
  CONSTRAINT Universal Joint : sm_lib/Joints/Universal Joint  SenseConstraintForce=on  SenseConstraintForceX=off  SenseConstraintForceY=off  SenseConstraintForceZ=off  SenseConstraintTorque=on  SenseConstraintTorqueX=off  SenseConstraintTorqueY=off  SenseConstraintTorqueZ=off  SenseTotalForce=off  SenseTotalForceX=off  SenseTotalForceY=off  SenseTotalForceZ=off  SenseTotalTorque=off  SenseTotalTorqueX=off  SenseTotalTorqueY=off  SenseTotalTorqueZ=off  CompositeWrenchDir=BaseOnFollower  CompositeWrenchFrame=BaseFrame  RxEquilibriumPosition=0  RxEquilibriumPositionUnits=deg  RxSpringStiffness=0  RxSpringStiffnessUnits=N*m/deg  RxDampingCoefficient=0  RxDampingCoefficientUnits=N*m/(deg/s)  RxTorqueActuationMode=NoTorque  RxMotionActuationMode=ComputedMotion  RxSensePosition=on  RxSenseVelocity=on  RxSenseAcceleration=on  RxSenseTorqueForce=off  RxPositionTargetSpecify=off  RxPositionTargetPriority=High  RxPositionTargetValue=0  RxPositionTargetValueUnits=deg  RxVelocityTargetSpecify=off  RxVelocityTargetPriority=High  RxVelocityTargetValue=0  RxVelocityTargetValueUnits=deg/s  RyEquilibriumPosition=0  RyEquilibriumPositionUnits=deg  RySpringStiffness=0  RySpringStiffnessUnits=N*m/deg  RyDampingCoefficient=0  RyDampingCoefficientUnits=N*m/(deg/s)  RyTorqueActuationMode=NoTorque  RyMotionActuationMode=ComputedMotion  RySensePosition=on  RySenseVelocity=on  RySenseAcceleration=on  RySenseTorqueForce=off  RyPositionTargetSpecify=off  RyPositionTargetPriority=High  RyPositionTargetValue=0  RyPositionTargetValueUnits=deg  RyVelocityTargetSpecify=off  RyVelocityTargetPriority=High  RyVelocityTargetValue=0  RyVelocityTargetValueUnits=deg/s
  Constant : Constant  Value=[0 0 0 0 0 0]
  Constant1 : Constant  Value=[0 0 0 0 0 0]
  Constant2 : Constant  Value=[0 0 0 0 0 0]
  Mux{,2..4} (4 alike) : Mux  Inputs=2
  Mux1 : Mux
  PS-Simulink Converter{1..5,7,9,11} (8 alike) : nesl_utility/PS-Simulink Converter  PhysicalDomain=network_engine_domain  SubClassName=ps_output  LeftPortType=input  RightPortType=output  PseudoPeriodic=off  Frequencies=[]  Unit=1  AffineConversion=off
  Rigid Transform (Position) : sm_lib/Frames and Transforms/Rigid Transform  TranslationMethod=Cartesian  TranslationStandardOffset=0  TranslationLengthUnit=m  TranslationStandardAxis=+Z  TranslationCartesianOffset=constraint.initDisp.initLinDisp+constraint.loc  TranslationROffset=0  TranslationROffsetUnits=m  TranslationZOffset=0  TranslationZOffsetUnits=m  TranslationThetaOffset=0  TranslationThetaOffsetUnits=deg  RotationMethod=None  RotationAngleUnits=rad  RotationStandardAxis=+Y  RotationAngle=0  RotationArbitraryAxis=[0 1 0]  FollAlignAxisA=+X  BaseAlignAxisA=+Y  FollAlignAxisB=+Y  BaseAlignAxisB=+Z  RotationSequenceAxes=FollowerAxes  RotationSequence=XYX  RotationSequenceAngles=[0 0 0]  RotationSequenceAnglesUnits=deg  RotationMatrix=[1 0 0; 0 1 0; 0 0 1]
  Rigid Transform (Position)1 : sm_lib/Frames and Transforms/Rigid Transform  TranslationMethod=Cartesian  TranslationStandardOffset=0  TranslationLengthUnit=m  TranslationStandardAxis=+Z  TranslationCartesianOffset=constraint.initDisp.initLinDisp+constraint.loc  TranslationROffset=0  TranslationROffsetUnits=m  TranslationZOffset=0  TranslationZOffsetUnits=m  TranslationThetaOffset=0  TranslationThetaOffsetUnits=deg  RotationMethod=None  RotationAngleUnits=rad  RotationStandardAxis=+Y  RotationAngle=0  RotationArbitraryAxis=[0 1 0]  FollAlignAxisA=+X  BaseAlignAxisA=+Y  FollAlignAxisB=+Y  BaseAlignAxisB=+Z  RotationSequenceAxes=FollowerAxes  RotationSequence=XYX  RotationSequenceAngles=[0 0 0]  RotationSequenceAnglesUnits=deg  RotationMatrix=[1 0 0; 0 1 0; 0 0 1]
  Rigid Transform (Orientation) : sm_lib/Frames and Transforms/Rigid Transform  TranslationMethod=None  TranslationStandardOffset=0  TranslationLengthUnit=m  TranslationStandardAxis=+Z  TranslationCartesianOffset=constraint.loc  TranslationROffset=0  TranslationROffsetUnits=m  TranslationZOffset=0  TranslationZOffsetUnits=m  TranslationThetaOffset=0  TranslationThetaOffsetUnits=deg  RotationMethod=RotationMatrix  RotationAngleUnits=rad  RotationStandardAxis=+Y  RotationAngle=0  RotationArbitraryAxis=[0 1 0]  FollAlignAxisA=+X  BaseAlignAxisA=+Y  FollAlignAxisB=+Y  BaseAlignAxisB=+Z  RotationSequenceAxes=FollowerAxes  RotationSequence=XYX  RotationSequenceAngles=[0 0 0]  RotationSequenceAnglesUnits=deg  RotationMatrix=constraint.orientation.rotationMatrix
  Rigid Transform (Orientation)1 : sm_lib/Frames and Transforms/Rigid Transform  TranslationMethod=None  TranslationStandardOffset=0  TranslationLengthUnit=m  TranslationStandardAxis=+Z  TranslationCartesianOffset=constraint.loc  TranslationROffset=0  TranslationROffsetUnits=m  TranslationZOffset=0  TranslationZOffsetUnits=m  TranslationThetaOffset=0  TranslationThetaOffsetUnits=deg  RotationMethod=RotationMatrix  RotationAngleUnits=rad  RotationStandardAxis=+Y  RotationAngle=0  RotationArbitraryAxis=[0 1 0]  FollAlignAxisA=+X  BaseAlignAxisA=+Y  FollAlignAxisB=+Y  BaseAlignAxisB=+Z  RotationSequenceAxes=FollowerAxes  RotationSequence=XYX  RotationSequenceAngles=[0 0 0]  RotationSequenceAnglesUnits=deg  RotationMatrix=constraint.orientation.rotationMatrix
  output : ToWorkspace  VariableName=constraint8_out  SaveFormat=Structure With Time  SampleTime=-1
  F : PMIOPort  Port=1  Side=Right
  B : PMIOPort  Port=2  Side=Left
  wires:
  PS-Simulink Converter4/1 -> Mux/2
  PS-Simulink Converter3/1 -> Mux/1
  Mux3/1 -> Assignment1/2
  Mux4/1 -> Assignment/2
  Constant/1 -> Assignment/1
  Constant1/1 -> Assignment1/1
  Constant2/1 -> Assignment2/1
  Assignment2/1 -> Mux1/3  "acceleration"
  Assignment1/1 -> Mux1/2  "velocity"
  Assignment/1 -> Mux1/1  "position"
  Mux/1 -> Mux1/4  "Constraint Forces"
  Mux1/1 -> output/1
  PS-Simulink Converter5/1 -> Mux2/2
  Mux2/1 -> Assignment2/2
  PS-Simulink Converter2/1 -> Mux3/2
  PS-Simulink Converter9/1 -> Mux3/1
  PS-Simulink Converter11/1 -> Mux4/2
  PS-Simulink Converter1/1 -> Mux4/1
  PS-Simulink Converter7/1 -> Mux2/1
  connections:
  Rigid Transform (Position)1/LConn1 -- F/RConn1
  Rigid Transform (Position)1/RConn1 -- Rigid Transform (Orientation)1/LConn1
  Rigid Transform (Orientation)/RConn1 -- CONSTRAINT Universal Joint/LConn1
  Rigid Transform (Position)/RConn1 -- Rigid Transform (Orientation)/LConn1
  Rigid Transform (Position)/LConn1 -- B/RConn1
  CONSTRAINT Universal Joint/RConn8 -- PS-Simulink Converter3/LConn1
  PS-Simulink Converter4/LConn1 -- CONSTRAINT Universal Joint/RConn9
  PS-Simulink Converter1/LConn1 -- CONSTRAINT Universal Joint/RConn2
  PS-Simulink Converter11/LConn1 -- CONSTRAINT Universal Joint/RConn5
  PS-Simulink Converter9/LConn1 -- CONSTRAINT Universal Joint/RConn3
  PS-Simulink Converter7/LConn1 -- CONSTRAINT Universal Joint/RConn4
  PS-Simulink Converter2/LConn1 -- CONSTRAINT Universal Joint/RConn6
  PS-Simulink Converter5/LConn1 -- CONSTRAINT Universal Joint/RConn7
  CONSTRAINT Universal Joint/RConn1 -- Rigid Transform (Orientation)1/RConn1
